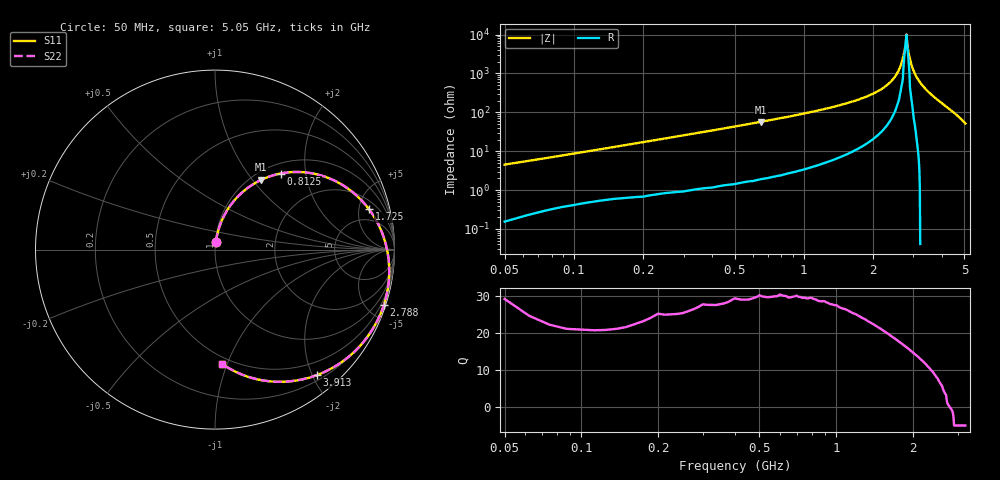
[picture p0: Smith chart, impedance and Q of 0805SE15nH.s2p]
! AVX Thin Film Operation		Date: May 2002
! Description: Accu-L® Series, Thin Film, SMD, RF Inductors
! Part Number: L0805150GEWTR
! 50 MHz  -  5.05 GHz
! Serial Measurements
# mhz S db R 50
!	S11		S21		S12		S22
!	dB	Phase	dB	Phase	dB	Phase	dB	Phase
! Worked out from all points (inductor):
!   401 points, 50 MHz to 5.05 GHz, reference 50 ohm
!   read as one part in series: L = 13.8 nH near 75 MHz
!   highest Q = 30 at 650 MHz (marker M1), where L = 13.9 nH
!   self-resonance near 2.775 GHz
!   S11 on the Smith chart (normalised r, x): 50 MHz: 1.01, +0.09; 812.5 MHz: 1.18, +1.45; 1.725 GHz: 3.01, +6.36; 2.788 GHz: 0.20, -6.29; 3.913 GHz: 0.28, -2.07; 5.05 GHz: 0.45, -0.96
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50  -27.35 84.1  -0.01 -2.7  -0.01 -2.7  -27.35 84.1
137.5  -19.14 80.1  -0.10 -7.1  -0.10 -7.1  -19.14 80.1
250  -14.16 74.9  -0.24 -12.7  -0.24 -12.7  -14.16 74.9
412.5  -10.09 67.3  -0.54 -20.5  -0.54 -20.5  -10.09 67.3
650  -6.62 56.4  -1.21 -31.4  -1.21 -31.4  -6.62 56.4
812.5  -5.05 49.3  -1.79 -38.4  -1.79 -38.4  -5.05 49.3
887.5  -4.46 46.1  -2.10 -41.6  -2.10 -41.6  -4.46 46.1
1262.5  -2.41 31.1  -3.99 -56.2  -3.99 -56.2  -2.41 31.1
1725  -1.04 14.7  -7.24 -71.9  -7.24 -71.9  -1.04 14.7
2200  -0.35 -0.5  -12.51 -85.7  -12.50 -85.7  -0.35 -0.5
2400  -0.20 -6.6  -16.13 -90.4  -16.10 -90.4  -0.20 -6.6
2550  -0.13 -11.1  -20.29 -92.4  -20.30 -92.4  -0.13 -11.1
2687.5  -0.10 -15.1  -27.25 -88.8  -27.20 -88.8  -0.10 -15.1
2787.5  -0.09 -18.1  -37.58 -17.6  -37.60 -17.6  -0.09 -18.1
2812.5  -0.09 -18.8  -37.40 0.8  -37.40 0.8  -0.09 -18.8
2887.5  -0.09 -21.0  -28.66 50.2  -28.70 50.2  -0.09 -21.0
3012.5  -0.12 -24.6  -21.62 62.1  -21.60 62.1  -0.12 -24.6
3162.5  -0.17 -28.9  -17.13 60.6  -17.10 60.6  -0.17 -28.9
3387.5  -0.31 -35.4  -13.07 56.0  -13.10 56.0  -0.31 -35.4
3912.5  -0.90 -50.8  -7.78 42.6  -7.78 42.6  -0.90 -50.8
4225  -1.46 -60.2  -5.81 34.2  -5.81 34.2  -1.46 -60.2
5050  -3.89 -86.3  -2.50 11.1  -2.50 11.1  -3.89 -86.3
